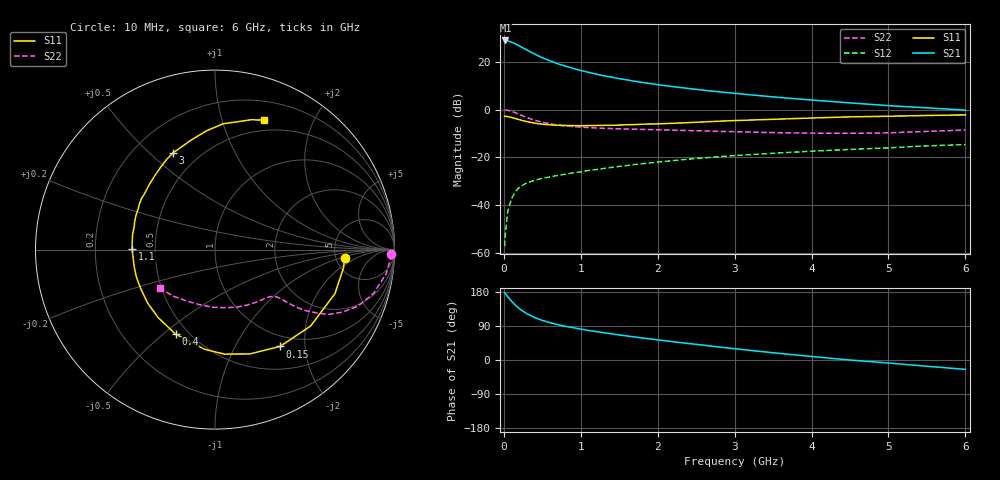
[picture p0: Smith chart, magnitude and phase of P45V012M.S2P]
! SIEMENS Small Signal Semiconductors
! BFP182
! Si NPN RF Bipolar Junction Transistor in SOT143
! VCE = 5 V  IC = 12 mA
! Common Emitter S-Parameters:  March  1996
# GHz  S  MA  R  50
!  f  S11  S21  S12  S22
! GHz  MAG  ANG  MAG  ANG  MAG  ANG  MAG  ANG
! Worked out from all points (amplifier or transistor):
!   36 points, 10 MHz to 6 GHz, reference 50 ohm
!   highest |S21| = 28.8 dB at 20 MHz (marker M1)
!   |S21| within 3 dB of that: start of sweep to 242.4 MHz
!   unconditionally stable (mu >= 1): 1.127 GHz to 5.42 GHz
!   at 250 MHz: K = 0.35, MSG = 28.6 dB, |S12| = -31.5 dB
!   at 1.4 GHz: K = 1.08, MAG = 17.1 dB, |S12| = -24.2 dB
!   at 6 GHz: K = 0.94, MSG = 7.2 dB, |S12| = -14.6 dB
!   S11 on the Smith chart (normalised r, x): 10 MHz: 5.98, -1.24; 150 MHz: 0.83, -1.55; 400 MHz: 0.43, -0.55; 1.1 GHz: 0.37, +0.00; 3 GHz: 0.36, +0.60; 6 GHz: 0.39, +1.38
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0.01  0.7237 -3.9  27.56 177.2  0.0014 79.3  0.9786 -1.5
0.02  0.7232 -8.0  27.69 175.0  0.0025 82.2  0.9792 -3.2
0.05  0.712 -20.1  27.14 167.2  0.0073 82.9  0.9628 -8.1
0.1  0.682 -38.6  25.46 155.4  0.0137 70.2  0.917 -15.4
0.15  0.6499 -56.1  23.55 144.8  0.0193 65.4  0.8562 -21.6
0.2  0.6133 -71.3  21.43 135.8  0.0235 60.3  0.7928 -26.0
0.25  0.5851 -84.7  19.29 128.3  0.0266 55.9  0.7331 -29.5
0.3  0.5581 -96.1  17.48 122.2  0.0293 52.8  0.6785 -31.6
0.4  0.5198 -115.0  14.4 112.1  0.0333 49.1  0.5986 -34.3
0.5  0.4937 -129.9  12.05 104.5  0.0367 46.8  0.5426 -35.5
0.6  0.4791 -141.6  10.42 98.5  0.0392 46.0  0.503 -36.1
0.7  0.4678 -152.0  9.028 93.4  0.042 46.1  0.4748 -36.5
0.8  0.4641 -160.3  8.06 89.0  0.0446 46.1  0.4546 -36.9
1  0.4584 -174.1  6.518 81.5  0.0499 46.8  0.4284 -37.8
1.1  0.4619 179.8  5.988 78.0  0.0534 46.7  0.4189 -38.6
1.5  0.4739 160.9  4.417 66.0  0.0649 47.0  0.3955 -42.4
2.2  0.516 135.0  3.005 48.2  0.0858 44.7  0.3708 -52.5
3  0.5878 113.3  2.181 29.8  0.109 39.3  0.3443 -68.2
3.5  0.6245 102.3  1.833 19.1  0.1219 35.3  0.3292 -79.7
4.5  0.7028 86.2  1.374 -0.1  0.1468 27.5  0.3187 -105.8
5.5  0.7507 74.5  1.083 -16.5  0.174 20.2  0.3497 -132.3
6  0.7719 69.1  0.971 -24.7  0.1852 15.4  0.3729 -145.0
